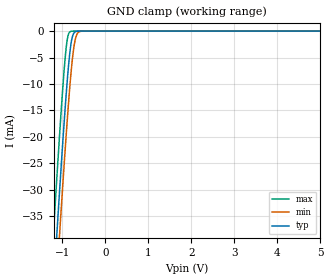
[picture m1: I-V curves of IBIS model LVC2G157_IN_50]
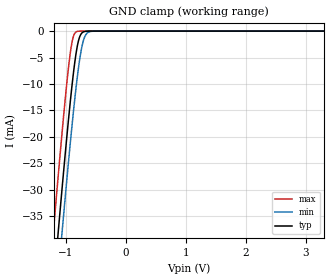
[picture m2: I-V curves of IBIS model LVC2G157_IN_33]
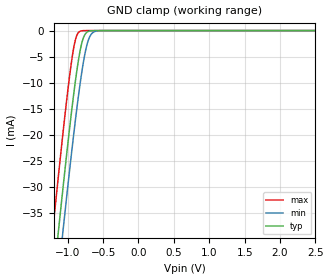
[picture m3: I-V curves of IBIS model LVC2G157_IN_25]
| TEXAS INSTRUMENTS INCORPORATED
| Standard Linear and Logic Group
| IBIS Model of SN74LVC2G157
| SINGLE 2-LINE TO 1-LINE DATA SELECTOR/MULTIPLEXER
| This file contains package information for the following:
|  SSOP 8-pin (DCT) package as [Component] LVC2G157_DCT
|  VSSOP 8-pin (DCU) package as [Component] LVC2G157_DCU
|  NanoStar WCSP 8-pin (YEA) package as [Component] LVC2G157_YEA
|  NanoFree WCSP 8-pin (YZA) package as [Component] LVC2G157_YZA
|  NanoStar WCSP 8-pin (YEP) package as [Component] LVC2G157_YEP
|  NanoFree WCSP 8-pin (YZP) package as [Component] LVC2G157_YZP
| This device can be powered at the following Vccs:
|  5 volt Vcc
|  3.3 volt Vcc
|  2.5 volt Vcc
|  1.8 volt Vcc
| This file provides unique models under the [Model Selector] for each Vcc.
| For operation at a specific Vcc, select the appropriate model after each
| [Model Selector] keyword.
[IBIS Ver]   3.2
[Comment char]  |_char
[File Name]   sn74lvc2g157.ibs
[File Rev]   1.2 | d_die
[Date]   September 03, 2003
[Source]   Data created from TI-SPICE simulations at TI-SLL.
[Notes]   The following is an IBIS list for the SN74LVC2G157.
   Please contact sllibis@ti.com with questions and
   comments concerning SLL IBIS models.
   - C_comp values are taken at a different test condition than
   the Ci in data sheet.
   - Power-clamp data has been deleted since there is no
   power-clamp diode in the device.
[Disclaimer] Property of Texas Instruments Incorporated. Unauthorized
   reproduction and/or distribution is strictly prohibited.
   This product is protected under copyright law.
   Created 2002,(C) Copyright 2002, Texas Instruments
   Incorporated, All Rights Reserved
   UNLESS THERE IS A SIGNED, WRITTEN AGREEMENT TO THE
   CONTRARY, TEXAS INSTRUMENTS (TI) IS PROVIDING THE IBIS
   MODELS AND WITHOUT ANY WARRANTY, EXPRESSED OR
   IMPLIED. TI assumes no liability for:
   1) the accuracy of the IBIS models provided to your
   company;
   2) the proper functioning of these IBIS Models in your
   design or for any resulting applications; or
   3) infringement of patents, copyrights or intellectual
   property rights resulting from your use of these IBIS
   models.
   TI provides IBIS Models as a service to our customers.
   You and your company shall not distribute, sell or give
   these models to anyone else without prior written
   permission from TI.
   TI reserves the right to make changes to our products or
   to discontinue any semiconductor product or service
   without notice, and advises our customers to obtain the
   latest version of relevant information to verify, before
   placing orders, that the information being relied on is
   current.
   Please be aware that your receipt and use of the IBIS
   information provided shall serve as acceptance of these
   terms and conditions. If you do not accept these terms,
   you should return or destroy the IBIS models and any
   other accompanying information immediately.
| Component LVC2G157_DCT 8-pin SSOP
[Component]   LVC2G157_DCT
[Manufacturer]   Texas Instruments, Inc.
[Package]
|   typ   min   max
R_pkg   2.900e-02   2.800e-02   3.100e-02
L_pkg   1.796e-09   1.666e-09   1.924e-09
C_pkg   1.090e-13   8.300e-14   1.360e-13
[Pin]   signal_name   model_name   R_pin   L_pin   C_pin
1   A   LVC2G157_IN   3.100e-02   1.894e-09   1.340e-13
2   B   LVC2G157_IN   2.800e-02   1.697e-09   8.600e-14
3   NY   LVC2G157_OUT   3.000e-02   1.722e-09   8.600e-14
4   GND   GND   3.000e-02   1.861e-09   1.300e-13
5   Y   LVC2G157_OUT   2.800e-02   1.924e-09   1.360e-13
6   NA_B   LVC2G157_IN   2.900e-02   1.736e-09   8.600e-14
7   NG   LVC2G157_IN   2.800e-02   1.666e-09   8.300e-14
8   VCC   POWER   3.000e-02   1.871e-09   1.320e-13
| Component LVC2G157_DCU 8-pin VSSOP
[Component]   LVC2G157_DCU
[Manufacturer]   Texas Instruments, Inc.
[Package]
|   typ   min   max
R_pkg   1.400e-02   1.300e-02   1.500e-02
L_pkg   1.289e-09   1.025e-09   2.014e-09
C_pkg   1.360e-13   6.600e-14   2.940e-13
[Pin]   signal_name   model_name   R_pin   L_pin   C_pin
1   A   LVC2G157_IN   1.400e-02   1.387e-09   1.760e-13
2   B   LVC2G157_IN   1.300e-02   1.026e-09   6.600e-14
3   NY   LVC2G157_OUT   1.300e-02   1.032e-09   6.700e-14
4   GND   GND   1.500e-02   2.014e-09   2.940e-13
5   Y   LVC2G157_OUT   1.400e-02   1.412e-09   1.780e-13
6   NA_B   LVC2G157_IN   1.300e-02   1.030e-09   6.600e-14
7   NG   LVC2G157_IN   1.300e-02   1.025e-09   6.600e-14
8   VCC   POWER   1.400e-02   1.386e-09   1.760e-13
| Component LVC2G157_YEA 8-pin NanoStar WCSP
[Component]   LVC2G157_YEA
[Manufacturer]   Texas Instruments, Inc.
[Package]
|   typ   min   max
R_pkg   0.001   0.001   0.001
L_pkg   0.021nH   0.021nH   0.021nH
C_pkg   0.043pF   0.042pF   0.044pF
[Pin]   signal_name   model_name   R_pin   L_pin   C_pin
1   A   LVC2G157_IN   0.046   2.861nH   0.321pF
2   B   LVC2G157_IN   0.037   2.437nH   0.286pF
3   NY   LVC2G157_OUT   0.034   2.419nH   0.286pF
4   GND   GND   0.043   2.784nH   0.321pF
5   Y   LVC2G157_OUT   0.043   2.784nH   0.321pF
6   NA_B   LVC2G157_IN   0.035   2.420nH   0.286pF
7   NG   LVC2G157_IN   0.037   2.437nH   0.286pF
8   VCC   POWER   0.046   2.860nH   0.321pF
| Component LVC2G157_YZA 8-pin NanoFree WCSP
[Component]   LVC2G157_YZA
[Manufacturer]   Texas Instruments, Inc.
[Package]
|   typ   min   max
R_pkg   0.001   0.001   0.001
L_pkg   0.021nH   0.021nH   0.021nH
C_pkg   0.043pF   0.042pF   0.044pF
[Pin]   signal_name   model_name   R_pin   L_pin   C_pin
1   A   LVC2G157_IN   0.046   2.861nH   0.321pF
2   B   LVC2G157_IN   0.037   2.437nH   0.286pF
3   NY   LVC2G157_OUT   0.034   2.419nH   0.286pF
4   GND   GND   0.043   2.784nH   0.321pF
5   Y   LVC2G157_OUT   0.043   2.784nH   0.321pF
6   NA_B   LVC2G157_IN   0.035   2.420nH   0.286pF
7   NG   LVC2G157_IN   0.037   2.437nH   0.286pF
8   VCC   POWER   0.046   2.860nH   0.321pF
| Component LVC2G157_YEP 8-pin NanoStar WCSP
[Component]   LVC2G157_YEP
[Manufacturer]   Texas Instruments, Inc.
[Package]
|   typ   min   max
R_pkg   0.001   0.001   0.001
L_pkg   0.021nH   0.021nH   0.021nH
C_pkg   0.043pF   0.042pF   0.044pF
[Pin]   signal_name   model_name   R_pin   L_pin   C_pin
1   A   LVC2G157_IN   0.046   2.861nH   0.321pF
2   B   LVC2G157_IN   0.037   2.437nH   0.286pF
3   NY   LVC2G157_OUT   0.034   2.419nH   0.286pF
4   GND   GND   0.043   2.784nH   0.321pF
5   Y   LVC2G157_OUT   0.043   2.784nH   0.321pF
6   NA_B   LVC2G157_IN   0.035   2.420nH   0.286pF
7   NG   LVC2G157_IN   0.037   2.437nH   0.286pF
8   VCC   POWER   0.046   2.860nH   0.321pF
| Component LVC2G157_YZP 8-pin NanoFree WCSP
[Component]   LVC2G157_YZP
[Manufacturer]   Texas Instruments, Inc.
[Package]
|   typ   min   max
R_pkg   0.001   0.001   0.001
L_pkg   0.021nH   0.021nH   0.021nH
C_pkg   0.043pF   0.042pF   0.044pF
[Pin]   signal_name   model_name   R_pin   L_pin   C_pin
1   A   LVC2G157_IN   0.046   2.861nH   0.321pF
2   B   LVC2G157_IN   0.037   2.437nH   0.286pF
3   NY   LVC2G157_OUT   0.034   2.419nH   0.286pF
4   GND   GND   0.043   2.784nH   0.321pF
5   Y   LVC2G157_OUT   0.043   2.784nH   0.321pF
6   NA_B   LVC2G157_IN   0.035   2.420nH   0.286pF
7   NG   LVC2G157_IN   0.037   2.437nH   0.286pF
8   VCC   POWER   0.046   2.860nH   0.321pF
| Model LVC2G157_IN
[Model Selector]   LVC2G157_IN
LVC2G157_IN_50   5 volt Vcc
LVC2G157_IN_33   3.3 volt Vcc
LVC2G157_IN_25   2.5 volt Vcc
LVC2G157_IN_18   1.8 volt Vcc
| Model LVC2G157_OUT
[Model Selector]   LVC2G157_OUT
LVC2G157_OUT_50   5 volt Vcc
LVC2G157_OUT_33   3.3 volt Vcc
LVC2G157_OUT_25   2.5 volt Vcc
LVC2G157_OUT_18   1.8 volt Vcc
| Models and submodels in the file (8): LVC2G157_IN_50 (Input), LVC2G157_IN_33 (Input), LVC2G157_IN_25 (Input), LVC2G157_IN_18 (Input), LVC2G157_OUT_50 (Output), LVC2G157_OUT_33 (Output), LVC2G157_OUT_25 (Output), LVC2G157_OUT_18 (Output)
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[Model]   LVC2G157_IN_50
Model_type  Input
Vinl=1.35
Vinh=3.85
| variable   typ   min   max
C_comp   3.21pF   2.51pF   4.33pF
[Temperature Range]   40   100   -40
| Ambient temperature   25   85   -40
[Voltage range]   5   4.5   5.5
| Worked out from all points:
|   GND clamp passes 1 mA (typ) near -0.77 V on its own axis
[GND Clamp]
| LVC2G157_IN_50
|   Voltage   I(typ)   I(min)   I(max)
-5V       -583.8mA   -590.8mA   -575.1mA
-1.21V    -48.93mA   -57.22mA   -38.3mA
-1.13V    -38.42mA   -46.71mA   -27.77mA
-1.07V    -30.71mA   -38.96mA   -20.13mA
-1.05V    -28.19mA   -36.42mA   -17.65mA
-915mV    -12.21mA   -19.95mA   -3.333mA
-870mV    -7.651mA   -14.9mA    -891.1uA
-815mV    -3.252mA   -9.299mA   -87.06uA
-770mV    -1.128mA   -5.445mA   -10.73uA
-705mV    -146.7uA   -1.723mA   -505nA
-575mV    -1.597uA   -52.97uA   -1.117nA
5V        9.69pA     12.83pA    9.218pA
[Model]   LVC2G157_IN_33
Model_type  Input
Vinl=0.8
Vinh=2.0
| variable   typ   min   max
C_comp   3.34pF   2.68pF   4.33pF
[Temperature Range]   40   100   -40
| Ambient temperature   25   85   -40
[Voltage range]   3.3   3   3.6
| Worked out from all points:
|   GND clamp passes 1 mA (typ) near -0.77 V on its own axis
[GND Clamp]
| LVC2G157_IN_33
|   Voltage   I(typ)   I(min)   I(max)
-3.3V     -341.5mA   -348.9mA   -332.3mA
-1.215V   -49.6mA    -57.88mA   -38.96mA
-1.185V   -45.62mA   -53.91mA   -34.98mA
-1.125V   -37.77mA   -46.06mA   -27.13mA
-1.065V   -30.08mA   -38.33mA   -19.51mA
-920mV    -12.75mA   -20.53mA   -3.718mA
-875mV    -8.124mA   -15.45mA   -1.065mA
-825mV    -3.922mA   -10.26mA   -137.1uA
-775mV    -1.291mA   -5.83mA    -13.57uA
-715mV    -205.4uA   -2.128mA   -808.5nA
-585mV    -2.266uA   -70.82uA   -1.783nA
3.3V      6.304pA    9.258pA    5.93pA
[Model]   LVC2G157_IN_25
Model_type  Input
Vinl=0.7
Vinh=1.7
| variable   typ   min   max
C_comp   3.42pF   2.81pF   4.39pF
[Temperature Range]   40   100   -40
| Ambient temperature   25   85   -40
[Voltage range]   2.5   2.3   2.7
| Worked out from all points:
|   GND clamp passes 1 mA (typ) near -0.77 V on its own axis
[GND Clamp]
| LVC2G157_IN_25
|   Voltage   I(typ)   I(min)   I(max)
-2.5V     -228.1mA   -235.8mA   -218.5mA
-1.23V    -51.59mA   -59.87mA   -40.97mA
-1.2V     -47.61mA   -55.9mA    -36.97mA
-1.13V    -38.42mA   -46.71mA   -27.77mA
-1.07V    -30.71mA   -38.96mA   -20.13mA
-925mV    -13.29mA   -21.11mA   -4.122mA
-880mV    -8.606mA   -15.99mA   -1.263mA
-830mV    -4.281mA   -10.75mA   -171.6uA
-780mV    -1.472mA   -6.227mA   -17.15uA
-720mV    -242.5uA   -2.354mA   -1.023uA
-600mV    -3.832uA   -109.2uA   -3.608nA
2.5V      4.713pA    7.577pA    4.389pA
